TYPE Alarm :
STRUCT
	//PRESSURE_Warning:BOOL;
	PRESSURE:BOOL;
	
	//MFC1_Warning:BOOL;
	MFC1:BOOL;
	
	//MFC2_Warning:BOOL;
	MFC2:BOOL;
	
	//MFC3_Warning:BOOL;
	MFC3:BOOL;
	
	//MFC4_Warning:BOOL;
	MFC4:BOOL;
	
	//MFC5_Warning:BOOL;
	MFC5:BOOL;
	
	//MFC6_Warning:BOOL;
	MFC6:BOOL;
	
	//MFC7_Warning:BOOL;
	MFC7:BOOL;
	
	//MFC8_Warning:BOOL;
	MFC8:BOOL;
	
	//MFC9_Warning:BOOL;
	MFC9:BOOL;
	
	//WALL_TEMP_Warning:BOOL;
	WALL_TEMP:BOOL;
	
	//LID_TEMP_Warning:BOOL;
	LID_TEMP:BOOL;
	
	//STAGE_TEMP_Warning:BOOL;
	STAGE_TEMP1:BOOL;
	STAGE_TEMP2:BOOL;
	STAGE_TEMP3:BOOL;
	STAGE_TEMP4:BOOL;
	
	

	Gas1FlowPressureOutOfRange:BOOL;
	Gas2FlowPressureOutOfRange:BOOL;
	Gas3FlowPressureOutOfRange:BOOL;
	Gas4FlowPressureOutOfRange:BOOL;
	Gas5FlowPressureOutOfRange:BOOL;
	Gas6FlowPressureOutOfRange:BOOL;
	Gas7FlowPressureOutOfRange:BOOL;
	Gas8FlowPressureOutOfRange:BOOL;
	Gas9FlowPressureOutOfRange:BOOL;	
	
	
	TurboN2PurgePressureOutOfRange:BOOL;
	PrepareTransferTimerout:BOOL;
	TransferWaferTimeout:BOOL;
	OpenGasValveTimeout:BOOL;
	CloseGasValveTimeout:BOOL;
	OpenCloseSlitValveTimeout:BOOL;
	ATMCheckTimeout:BOOL;
	
	PLC:BOOL;	
	DRY_PUMP:BOOL;
	PENDULUM_VALVE:BOOL;
	TURBO_PUMP:BOOL;
	
	//PROCESS TOLERANCE
	TOLERANCE_PRESSURE:BOOL;
	TOLERANCE_MFC1:BOOL;
	TOLERANCE_MFC2:BOOL;
	TOLERANCE_MFC3:BOOL;
	TOLERANCE_MFC4:BOOL;
	TOLERANCE_MFC5:BOOL;
	TOLERANCE_MFC6:BOOL;
	TOLERANCE_MFC7:BOOL;
	TOLERANCE_MFC8:BOOL;
	TOLERANCE_MFC9:BOOL;
	TOLERANCE_WALL_TEMP:BOOL;
	TOLERANCE_LID_TEMP:BOOL;
	TOLERANCE_STAGE_TEMP1,
	TOLERANCE_STAGE_TEMP2,
	TOLERANCE_STAGE_TEMP3,
	TOLERANCE_STAGE_TEMP4: BOOL;


	
END_STRUCT
END_TYPE
